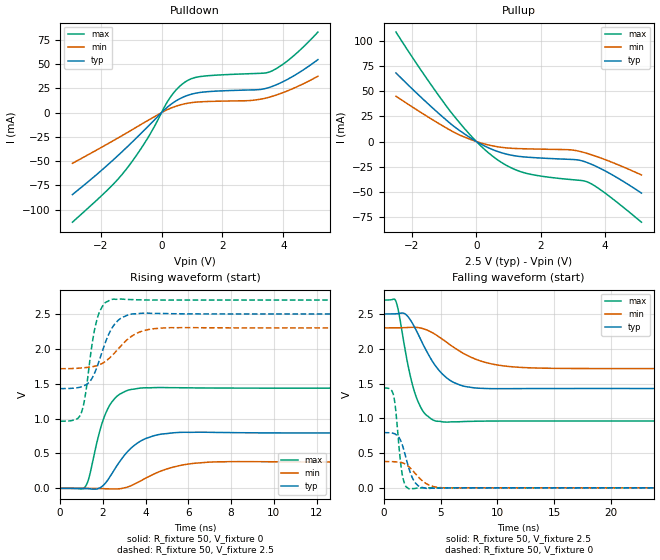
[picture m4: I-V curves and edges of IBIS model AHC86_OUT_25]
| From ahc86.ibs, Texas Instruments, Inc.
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[Model]   AHC86_OUT_25
Model_type  Output
|Vref =   0
|Rref =   500
Cref =   50p
Vmeas =   1.25
| variable   typ   min   max
C_comp   12.34pF   10.56pF   14.77pF
| C_pullup   11.77pF   10.56pF   13.28pF
| C_pulldown   12.90pF   11.51pF   14.77pF
[Temperature Range]   40   100   -40
| Ambient temperature   25   85   -40
[Voltage range]   2.5   2.3   2.7
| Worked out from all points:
|   slope of the pulldown table from 0 to 0.375 V, typ, clamps not added: 37.2 ohm
|   slope of the pullup table from 0 to 0.375 V, typ, clamps not added: 59.9 ohm
|   rising waveform, R_fixture 50, V_fixture 0: 20-80 % time 1.24ns typ, 1.7ns min, 788ps max; typ from 0 V to 0.794 V
|   falling waveform, R_fixture 50, V_fixture 2.5: 20-80 % time 2.33ns typ, 3.63ns min, 1.35ns max; typ from 2.5 V to 1.43 V
|   rising waveform, R_fixture 50, V_fixture 2.5: 20-80 % time 805ps typ, 1.19ns min, 503ps max; typ from 1.43 V to 2.5 V
|   falling waveform, R_fixture 50, V_fixture 0: 20-80 % time 885ps typ, 1.38ns min, 508ps max; typ from 0.794 V to 0 V
[Pulldown]
| AHC86_OUT_25
|   Voltage   I(typ)   I(min)   I(max)
-2.925V   -84.52mA   -52.28mA   -113mA
-1.8V     -54.82mA   -32.75mA   -80.62mA
-1.205V   -37.64mA   -22.04mA   -60.28mA
-490mV    -15.69mA   -8.829mA   -28.09mA
265mV     7.52mA     4.123mA    14.76mA
685mV     15.66mA    8.561mA    29.57mA
965mV     18.91mA    10.25mA    34.83mA
1.295V    20.97mA    11.21mA    37.35mA
2.885V    23.41mA    12.43mA    40.19mA
3.535V    25.98mA    15.9mA     41.87mA
4.285V    36.92mA    24.43mA    57.2mA
5.135V    54.7mA     37.55mA    83.12mA
[Pullup]
| AHC86_OUT_25
|   Voltage   I(typ)   I(min)   I(max)
-2.5V     68.34mA    45.17mA    109.1mA
-1.595V   40.37mA    26.34mA    65.2mA
-805mV    17.87mA    11.17mA    29.92mA
-120mV    2.341mA    1.34mA     4.04mA
475mV     -7.653mA   -4.114mA   -13.84mA
985mV     -12.92mA   -6.478mA   -24.64mA
1.47V     -15.3mA    -7.208mA   -30.97mA
2.885V    -17.76mA   -8.179mA   -37.75mA
3.21V     -18.66mA   -9.781mA   -38.67mA
3.48V     -21.39mA   -12.2mA    -40.65mA
4.085V    -30.69mA   -19.02mA   -53.35mA
5.135V    -51.41mA   -33.33mA   -80.43mA
[Ramp]
| AHC86_OUT_25
| variable   typ   min   max
dV/dt_r   0.49/1.30E-09   0.23/1.80E-09   0.87/8.21E-10
dV/dt_f   0.65/2.40E-09   0.36/3.74E-09   1.06/1.41E-09
R_load = 50
[Rising Waveform]
| AHC86_OUT_25
R_fixture =   50
C_fixture =   0
L_fixture =   0
V_fixture =   0
V_fixture_min = 0
V_fixture_max = 0
|   Time   V(typ)   V(min)   V(max)
0s        -66.56uV   -57.66uV   -52.66uV
1.155ns   -2.586mV   -720.4uV   15.08mV
1.355ns   -5.91mV    -993uV     157.7mV
1.93ns    19.85mV    -3.755mV   902.2mV
2.3ns     151.8mV    -7.932mV   1.181V
2.805ns   390.5mV    -5.005mV   1.353V
3.8ns     683.8mV    111.6mV    1.439V
5.335ns   796.9mV    307.6mV    1.443V
7.365ns   801.3mV    380mV      1.438V
50ns      793.7mV    377.6mV    1.436V
[Falling Waveform]
| AHC86_OUT_25
R_fixture =   50
C_fixture =   0
L_fixture =   0
V_fixture =   2.5
V_fixture_min = 2.3
V_fixture_max = 2.7
|   Time   V(typ)   V(min)   V(max)
0s        2.5V       2.3V       2.7V
1.06ns    2.502V     2.3V       2.686V
1.35ns    2.506V     2.301V     2.497V
1.925ns   2.495V     2.304V     1.946V
2.785ns   2.288V     2.307V     1.34V
3.555ns   2.032V     2.283V     1.079V
4.605ns   1.742V     2.198V     959.9mV
6.99ns    1.464V     1.934V     953.1mV
11.87ns   1.427V     1.733V     961mV
50ns      1.429V     1.715V     961.9mV
[Rising Waveform]
| AHC86_OUT_25
R_fixture =   50
C_fixture =   0
L_fixture =   0
V_fixture =   2.5
V_fixture_min = 2.3
V_fixture_max = 2.7
|   Time   V(typ)   V(min)   V(max)
0s        1.429V     1.715V     961.9mV
960ps     1.452V     1.725V     1.058V
1.155ns   1.477V     1.73V      1.292V
1.515ns   1.591V     1.745V     2.109V
1.735ns   1.748V     1.76V      2.433V
2.055ns   2.037V     1.806V     2.644V
2.475ns   2.322V     1.918V     2.712V
3.605ns   2.504V     2.226V     2.703V
5.08ns    2.505V     2.303V     2.7V
50ns      2.5V       2.3V       2.7V
[Falling Waveform]
| AHC86_OUT_25
R_fixture =   50
C_fixture =   0
L_fixture =   0
V_fixture =   0
V_fixture_min = 0
V_fixture_max = 0
|   Time   V(typ)   V(min)   V(max)
0s        793.7mV    377.6mV    1.436V
845ps     783.5mV    375.9mV    1.342V
1.04ns    769.8mV    374.5mV    1.14V
1.415ns   704.5mV    368.7mV    467.2mV
1.625ns   621mV      360.9mV    197.3mV
1.905ns   463.3mV    341.2mV    30.81mV
2.29ns    240.8mV    292.3mV    -18.41mV
3.185ns   13.85mV    133.3mV    -1.543mV
5.345ns   -1.891mV   -593.7uV   -41.84uV
50ns      -63.13uV   -57.59uV   -48.86uV
